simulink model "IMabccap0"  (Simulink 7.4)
settings: Solver=ode45  StartTime=0.0  StopTime=2.5  RelTol=1e-3
InitFcn:
  | imparamcap0
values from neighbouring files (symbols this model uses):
  Bm = 0.10    (= 0.1)    [IMabc2.m]    (also in imabcparam.m = 0.01; IMabcrun0.m = 0.01; IMabcrun1.m = 0.001; IMcur0.m = 1e-06)
  D = str2num(get(h,'string'))    [acttrcalc1.m]
  J = 0.02    [imabcparam.m]    (also in IMabcrun0.m; IMabcrun1.m; imdefSIvec1.m = 0.03)
  Lm = eval(get(hLm,'String'))    [im3d.m]    (also in IMabc2.m = 4.5; imabcparam.m = 0.0847; IMabcrun0.m = 0.0847; IMabcrun1.m = 0.0847)
  Lrr = [Lr   -Lm/2 -Lm/2    [IMabc2.m]    (also in IMabcf0.m = [Lr   -Lm1/2 -Lm1/2; IMabcf1.m = [Lr   -Lm1/2 -Lm1/2)
  Lss = [Ls   -Lm/2 -Lm/2    [IMabc2.m]    (also in IMabcf0.m = [Ls   -Lm1/2 -Lm1/2; IMabcf1.m = [Ls   -Lm1/2 -Lm1/2)
  nsync = 120*freq0/p    (= 1800)    [imabcparam.m]
  p = cos(beta-alpha)    [abcRwdg.m]    (also in alternator.m = 0:pi/20:2*pi; altwdgs.m = 0:pi/20:2*pi; brushlessdcB.m = 0:pi/100:2*pi; brushlessdcnew.m = 0:pi/100:2*pi)
  R = str2num(get(h,'string'))    [acttrcalc1.m]    (also in IMabc2.m = diag([Rs Rs Rs Rr Rr Rr]); IMabcf0.m = diag([Rs Rs Rs Rr Rr Rr]); IMabcf1.m = diag([Rs Rs Rs Rr Rr Rr]); IMcurf0.m = diag([Rs Rs Rr Rr]))
  Vm = Vll*sqrt(2/3)    [imabcparam.m]
  wo = 2*pi*freq0    [calc0.m]    (also in IMabc2.m = 376.991118431; imabcparam.m = 376.991118431; IMabcrun0.m = 376.991118431; IMabcrun1.m = 376.991118431)
undefined symbols (not defined in the file or in its folder): Row, vector

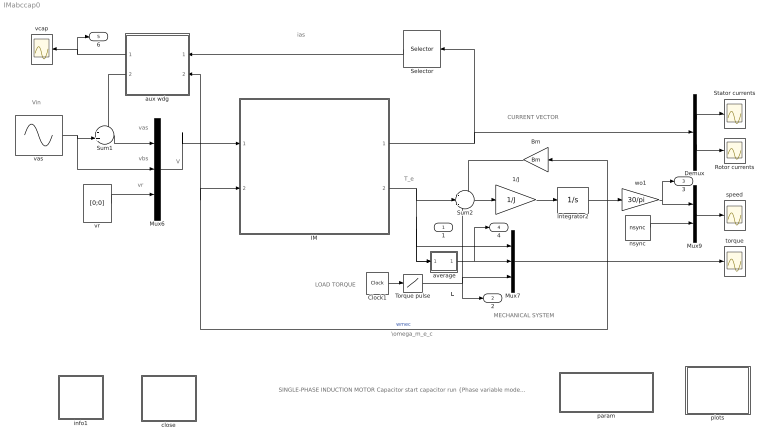
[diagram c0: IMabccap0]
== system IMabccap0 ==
  note: LOAD TORQUE
  note: T_L
  note: SINGLE-PHASE INDUCTION MOTOR Capacitor start capacitor run {Phase variable model} [SI]
  note: T_e
  note: I
  note: MECHANICAL SYSTEM
  note: \omega_m_e_c
  note: CURRENT VECTOR
  note: V
  note: vas
  note: vbs
  note: vr
  note: ias
  note: Vin
  " average" : Subsystem
  1/J : Gain  Gain=1/J  ParameterDataType=sfix(16)  ParameterScaling=2^0  OutDataType=sfix(16)  OutScaling=2^0
  Bm : Gain  Gain=Bm  ParameterDataType=sfix(16)  ParameterScaling=2^0  OutDataType=sfix(16)  OutScaling=2^0
  Clock1 : Clock
  Demux : Demux  Outputs=2
  IM : Subsystem
  Integrator2 : Integrator
  Mux6 : Mux  Inputs=3
  Mux7 : Mux  Inputs=3
  Mux9 : Mux  Inputs=2
  Rotor currents : Scope
  Selector : Selector  InputPortWidth=4  IndexOptions=Index vector (dialog)  Indices=[1]  OutputSizes=1
  Stator currents : Scope
  Sum1 : Sum  Inputs=-+|  OutDataType=sfix(16)  OutScaling=2^0
  Sum2 : Sum  Inputs=-+-  OutDataType=sfix(16)  OutScaling=2^0
  Torque pulse : Lookup  InputValues=[0 1 1 1.5 1.5 2]  Table=[0 0 2 2 3 3]  OutDataType=sfix(16)  OutScaling=2^0
  aux wdg : Subsystem  mask{Cstart=183e-6, Crun=30e-6, p=4, Nsw=3/4}
      mask prompts: Cstart "Start capacitance [F]"; Crun "Run capacitance [F}"; p "Number of poles"; Nsw "Speed when switch disconnects [pu]"
  close : Subsystem
  info1 : Subsystem
  nsync : Constant  Value=nsync  OutDataType=sfix(16)  OutScaling=2^0
  param : Subsystem
  plots : Subsystem
  speed : Scope
  torque : Scope
  vas : Sin  Amplitude=Vm  Bias=0  Frequency=wo  Phase=pi/2  Samples=10  SampleTime=0
  vcap : Scope
  vr : Constant  Value=[0;0]  VectorParams1D=off  OutDataType=sfix(16)  OutScaling=2^0
  wo1 : Gain  Gain=30/pi  ParameterDataType=sfix(16)  ParameterScaling=2^0  OutDataType=sfix(16)  OutScaling=2^0
  1 : Outport
  2 : Outport  Port=2
  3 : Outport  Port=3
  4 : Outport  Port=4
  6 : Outport  Port=5
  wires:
  Demux/1 -> Stator currents/1
  Demux/2 -> Rotor currents/1
  IM/1(I) -> Demux/1, Selector/1
  Sum2/1 -> 1/J/1
  1/J/1 -> Integrator2/1
  Mux9/1 -> speed/1
  Integrator2/1 -> wo1/1, Bm/1, IM/2(wmec), aux wdg/2(wmec)  "wmec"
  Mux7/1 -> torque/1
  Clock1/1 -> Torque pulse/1
  IM/2(Te) -> Sum2/2, Mux7/1, " average"/1(sig), 1/1
  nsync/1 -> Mux9/2
  Bm/1 -> Sum2/1
  wo1/1 -> Mux9/1, 3/1
  Torque pulse/1 -> Sum2/3, 2/1, Mux7/3
  vr/1 -> Mux6/3
  vas/1 -> Mux6/2, Sum1/2
  Selector/1 -> aux wdg/1(ias)
  Sum1/1 -> Mux6/1
  aux wdg/2(vaux) -> Sum1/1
  aux wdg/1(vcap) -> vcap/1, 6/1
  Mux6/1 -> IM/1(V)
  " average"/1(ave) -> Mux7/2, 4/1

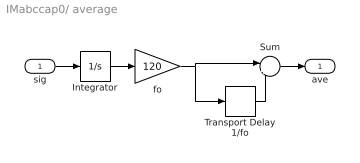
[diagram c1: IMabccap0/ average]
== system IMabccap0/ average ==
  sig : Inport  OutDataType=sfix(16)  OutScaling=2^0
  Integrator : Integrator
  Sum : Sum  Inputs=|+-  OutDataType=sfix(16)  OutScaling=2^0
  Transport Delay 1/fo : TransportDelay  DelayTime=1/120
  fo : Gain  Gain=120  ParameterDataType=sfix(16)  ParameterScaling=2^0  OutDataType=sfix(16)  OutScaling=2^0
  ave : Outport
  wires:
  Sum/1 -> ave/1
  Transport Delay 1/fo/1 -> Sum/2
  sig/1 -> Integrator/1
  fo/1 -> Transport Delay 1/fo/1, Sum/1
  Integrator/1 -> fo/1

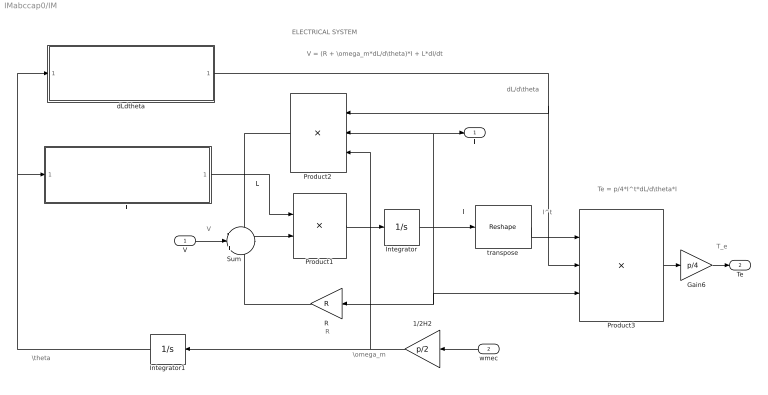
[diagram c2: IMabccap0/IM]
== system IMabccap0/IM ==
  note: I
  note: I^t
  note: ELECTRICAL SYSTEM
  note: V
  note: \omega_m
  note: \theta
  note: L
  note: T_e
  note: dL/d\theta
  note: R
  note: V = (R + \omega_m*dL/d\theta)*I + L*dI/dt
  note: Te = p/4*I^t*dL/d\theta*I
  V : Inport  OutDataType=sfix(16)  OutScaling=2^0
  wmec : Inport  Port=2  OutDataType=sfix(16)  OutScaling=2^0
  1/2H2 : Gain  Gain=p/2  ParameterDataType=sfix(16)  ParameterScaling=2^0  OutDataType=sfix(16)  OutScaling=2^0
  Gain6 : Gain  Gain=p/4  ParameterDataType=sfix(16)  ParameterScaling=2^0  OutDataType=sfix(16)  OutScaling=2^0
  Integrator : Integrator  InitialCondition=[0 ;0 ;0; 0 ]
  Integrator1 : Integrator
  L : Subsystem
  Product1 : Product  Inputs=/*  Multiplication=Matrix(*)  OutDataType=sfix(16)  OutScaling=2^0
  Product2 : Product  Inputs=***  Multiplication=Matrix(*)  OutDataType=sfix(16)  OutScaling=2^0
  Product3 : Product  Inputs=3  Multiplication=Matrix(*)  OutDataType=sfix(16)  OutScaling=2^0
  R : Gain  Gain=R  Multiplication=Matrix(K*u)  ParameterDataType=sfix(16)  ParameterScaling=2^0  OutDataType=sfix(16)  OutScaling=2^0
  Sum : Sum  Inputs=-|+|-  OutDataType=sfix(16)  OutScaling=2^0
  dLdtheta : Subsystem
  transpose : Reshape  OutputDimensionality=Row vector (2-D)  OutputDimensions=[1,6]
  I : Outport
  Te : Outport  Port=2
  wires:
  Product1/1 -> Integrator/1
  Integrator/1 -> Product3/3, R/1, transpose/1, Product2/2, I/1
  Sum/1 -> Product1/2
  R/1 -> Sum/3
  transpose/1 -> Product3/1
  Product2/1 -> Sum/1
  dLdtheta/1(dLdtheta) -> Product3/2, Product2/1
  Product3/1 -> Gain6/1
  1/2H2/1 -> Integrator1/1, Product2/3
  Integrator1/1 -> dLdtheta/1(theta1), L/1(theta)
  L/1(L) -> Product1/1
  V/1 -> Sum/2
  Gain6/1 -> Te/1
  wmec/1 -> 1/2H2/1

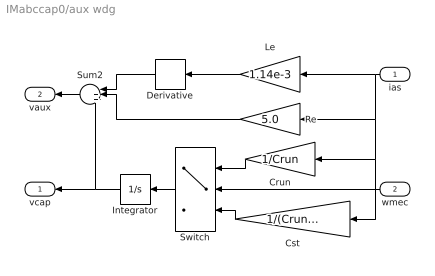
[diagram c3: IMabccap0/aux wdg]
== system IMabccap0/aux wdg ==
  ias : Inport  OutDataType=sfix(16)  OutScaling=2^0
  wmec : Inport  Port=2  OutDataType=sfix(16)  OutScaling=2^0
  Crun : Gain  Gain=1/Crun  ParameterDataType=sfix(16)  ParameterScaling=2^0  OutDataType=sfix(16)  OutScaling=2^0
  Cst : Gain  Gain=1/(Crun+Cstart)  ParameterDataType=sfix(16)  ParameterScaling=2^0  OutDataType=sfix(16)  OutScaling=2^0
  Derivative : Derivative
  Integrator : Integrator
  Le : Gain  Gain=1.14e-3  ParameterDataType=sfix(16)  ParameterScaling=2^0  OutDataType=sfix(16)  OutScaling=2^0
  Re : Gain  Gain=5.0  ParameterDataType=sfix(16)  ParameterScaling=2^0  OutDataType=sfix(16)  OutScaling=2^0
  Sum2 : Sum  Inputs=|+++  OutDataType=sfix(16)  OutScaling=2^0
  Switch : Switch  Threshold=Nsw*377*2/p
  vcap : Outport
  vaux : Outport  Port=2
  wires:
  ias/1 -> Le/1, Crun/1, Cst/1, Re/1
  wmec/1 -> Switch/2
  Integrator/1 -> vcap/1, Sum2/3
  Sum2/1 -> vaux/1
  Switch/1 -> Integrator/1
  Crun/1 -> Switch/1
  Cst/1 -> Switch/3
  Re/1 -> Sum2/2
  Derivative/1 -> Sum2/1
  Le/1 -> Derivative/1

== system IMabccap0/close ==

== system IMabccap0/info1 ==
  note: This demo simulates the starting characteristics of a capacitor- start capacitor-run single-phase induction motor. A dq version of this case is given in file .

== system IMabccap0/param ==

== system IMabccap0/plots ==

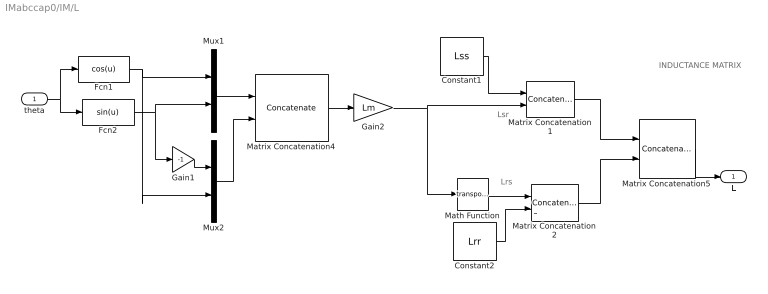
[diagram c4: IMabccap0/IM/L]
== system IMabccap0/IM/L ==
  note: L
  note: INDUCTANCE MATRIX
  note: Lsr
  note: Lrs
  theta : Inport  OutDataType=sfix(16)  OutScaling=2^0
  Constant1 : Constant  Value=Lss  VectorParams1D=off  OutDataType=sfix(16)  OutScaling=2^0
  Constant2 : Constant  Value=Lrr  VectorParams1D=off  OutDataType=sfix(16)  OutScaling=2^0
  Fcn1 : Fcn  Expr=cos(u)
  Fcn2 : Fcn  Expr=sin(u)
  Gain1 : Gain  Gain=-1  ParameterDataType=sfix(16)  ParameterScaling=2^0  OutDataType=sfix(16)  OutScaling=2^0
  Gain2 : Gain  Gain=Lm  ParameterDataType=sfix(16)  ParameterScaling=2^0  OutDataType=sfix(16)  OutScaling=2^0
  Math Function : Math  Operator=transpose
  Matrix Concatenation1 : Concatenate  Mode=Multidimensional array  ConcatenateDimension=2
  Matrix Concatenation2 : Concatenate  Mode=Multidimensional array  ConcatenateDimension=2
  Matrix Concatenation4 : Concatenate  Mode=Multidimensional array  ConcatenateDimension=2
  Matrix Concatenation5 : Concatenate  Mode=Multidimensional array
  Mux1 : Mux  Inputs=2
  Mux2 : Mux  Inputs=2
  L : Outport
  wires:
  Matrix Concatenation5/1 -> L/1
  theta/1 -> Fcn1/1, Fcn2/1
  Math Function/1 -> Matrix Concatenation2/1
  Gain2/1 -> Matrix Concatenation1/2, Math Function/1
  Mux1/1 -> Matrix Concatenation4/1
  Matrix Concatenation4/1 -> Gain2/1
  Matrix Concatenation1/1 -> Matrix Concatenation5/1
  Matrix Concatenation2/1 -> Matrix Concatenation5/2
  Constant1/1 -> Matrix Concatenation1/1
  Constant2/1 -> Matrix Concatenation2/2
  Fcn2/1 -> Mux1/2, Gain1/1
  Fcn1/1 -> Mux1/1, Mux2/2
  Gain1/1 -> Mux2/1
  Mux2/1 -> Matrix Concatenation4/2

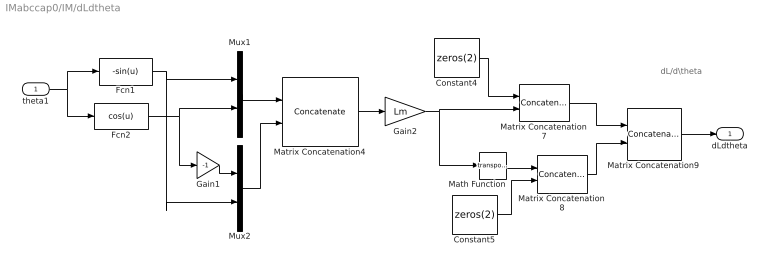
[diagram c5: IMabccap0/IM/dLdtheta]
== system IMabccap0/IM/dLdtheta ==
  note: dL/d\theta
  theta1 : Inport  OutDataType=sfix(16)  OutScaling=2^0
  Constant4 : Constant  Value=zeros(2)  VectorParams1D=off  OutDataType=sfix(16)  OutScaling=2^0
  Constant5 : Constant  Value=zeros(2)  VectorParams1D=off  OutDataType=sfix(16)  OutScaling=2^0
  Fcn1 : Fcn  Expr=-sin(u)
  Fcn2 : Fcn  Expr=cos(u)
  Gain1 : Gain  Gain=-1  ParameterDataType=sfix(16)  ParameterScaling=2^0  OutDataType=sfix(16)  OutScaling=2^0
  Gain2 : Gain  Gain=Lm  ParameterDataType=sfix(16)  ParameterScaling=2^0  OutDataType=sfix(16)  OutScaling=2^0
  Math Function : Math  Operator=transpose
  Matrix Concatenation4 : Concatenate  Mode=Multidimensional array  ConcatenateDimension=2
  Matrix Concatenation7 : Concatenate  Mode=Multidimensional array  ConcatenateDimension=2
  Matrix Concatenation8 : Concatenate  Mode=Multidimensional array  ConcatenateDimension=2
  Matrix Concatenation9 : Concatenate  Mode=Multidimensional array
  Mux1 : Mux  Inputs=2
  Mux2 : Mux  Inputs=2
  dLdtheta : Outport
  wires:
  Matrix Concatenation9/1 -> dLdtheta/1
  Matrix Concatenation7/1 -> Matrix Concatenation9/1
  Matrix Concatenation8/1 -> Matrix Concatenation9/2
  Constant4/1 -> Matrix Concatenation7/1
  Constant5/1 -> Matrix Concatenation8/2
  Math Function/1 -> Matrix Concatenation8/1
  Mux1/1 -> Matrix Concatenation4/1
  Matrix Concatenation4/1 -> Gain2/1
  Fcn2/1 -> Mux1/2, Gain1/1
  Fcn1/1 -> Mux1/1, Mux2/2
  Gain1/1 -> Mux2/1
  Mux2/1 -> Matrix Concatenation4/2
  theta1/1 -> Fcn1/1, Fcn2/1
  Gain2/1 -> Matrix Concatenation7/2, Math Function/1
